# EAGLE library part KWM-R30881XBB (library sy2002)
8x8 LED Matrix Display KWM-R30881ABB KWM-R30881CBB
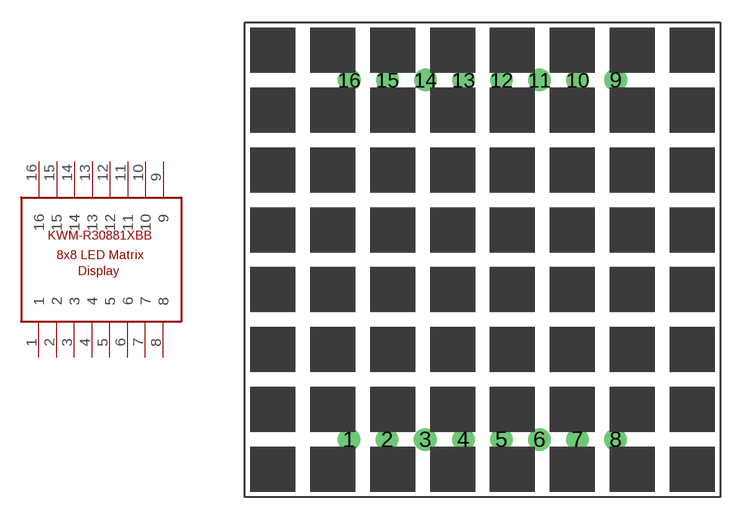
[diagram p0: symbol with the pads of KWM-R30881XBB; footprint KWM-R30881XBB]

Designator prefix -

## KWM-R30881XBB  [KWM-R30881XBB]
1  1
2  2
3  3
4  4
5  5
6  6
7  7
8  8
9  9
10  10
11  11
12  12
13  13
14  14
15  15
16  16

## Footprint KWM-R30881XBB (pad centres in mm)
drill 1: 1 -8.9,-12; 2 -6.36,-12; 3 -3.82,-12; 4 -1.28,-12; 5 1.26,-12; 6 3.8,-12; 7 6.34,-12; 8 8.88,-12; 9 8.89,12; 10 6.35,12; 11 3.81,12; 12 1.27,12; 13 -1.27,12; 14 -3.81,12; 15 -6.35,12; 16 -8.89,12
